FUNCTION FC 54 : VOID
TITLE =COPY DATA FROM OP_37 A PLC
AUTHOR : Davi
VERSION : 0.1

BEGIN
NETWORK
TITLE =ASPO (REEL)

      UN    M     47.1;
      SPB   ASP1;
      SPA   ASP2;

ASP1: L     DB14.DBD  286;
      T     DB14.DBD   52;
      L     DB14.DBD  290;
      T     DB14.DBD   56;

ASP2: NOP   0;

NETWORK
TITLE =STRAIGHTENER

      UN    M     47.2;
      SPB   SPI1;
      SPA   SPI2;

SPI1: L     DB14.DBD  294;
      T     DB14.DBD  150;
      L     DB14.DBD  298;
      T     DB14.DBD   48;
      L     DB14.DBD  302;
      T     DB14.DBD   24;
      L     DB14.DBD  306;
      T     DB14.DBD   44;

SPI2: NOP   0;

NETWORK
TITLE =HANDLING PROGRAM > WORKING AREA

      U     M     47.3;
      U     E     56.7;
      SPB   HAND;
      SPA   NOTH;

HAND: L     DB16.DBD  290;
      T     DB14.DBD  290;

      L     DB16.DBD   52;
      T     DB14.DBD   52;

      L     DB16.DBD  150;
      T     DB14.DBD  150;

      L     DB16.DBD   48;
      T     DB14.DBD   48;

      L     DB16.DBD   24;
      T     DB14.DBD   24;

      L     DB16.DBD   44;
      T     DB14.DBD   44;

      L     DB16.DBD  266;
      T     DB14.DBD  134;

      L     DB16.DBD  270;
      T     DB14.DBD  138;

      L     DB16.DBD  274;
      T     DB14.DBD  282;

      L     DB16.DBD  278;
      T     DB14.DBD  142;

NOTH: NOP   0;



END_FUNCTION

